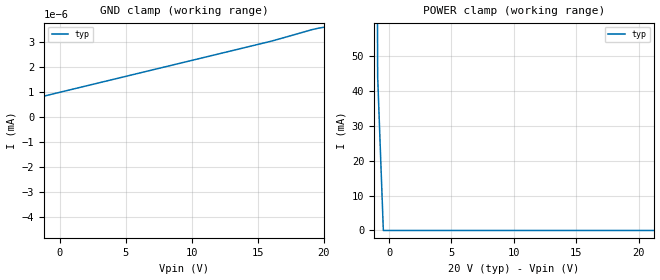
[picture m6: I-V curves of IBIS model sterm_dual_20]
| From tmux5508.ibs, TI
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| sterm_dual_20
[Model]   sterm_dual_20
Model_type   Terminator
|   typ   min   max
C_comp   2.533030e-12   NA   NA
[Voltage Range]   20   NA   NA
[Temperature Range]   27   NA   NA
[Power Clamp Reference]   20   NA   NA
[GND Clamp Reference]   0   NA   NA
[GND Clamp]
|   Voltage   I(typ)   I(min)   I(max)
-25V      -2.839A    NA         NA
-20.45V   -1.081uA   NA         NA
-20V      -1.588nA   NA         NA
-15.91V   -1.034nA   NA         NA
15.91V    3.008nA    NA         NA
19.09V    3.479nA    NA         NA
20V       3.577nA    NA         NA
[POWER Clamp]
|   Voltage   I(typ)   I(min)   I(max)
-5V       6.669A     NA         NA
-1.364V   578.8mA    NA         NA
-909.1mV  44.16mA    NA         NA
-454.5mV  669.9nA    NA         NA
40V       -4.292nA   NA         NA
